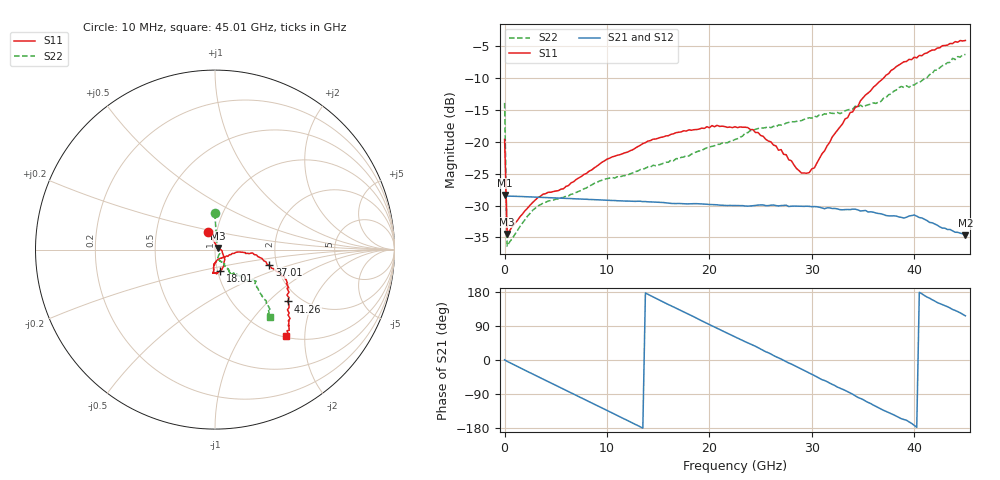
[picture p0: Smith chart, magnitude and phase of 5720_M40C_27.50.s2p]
! Device:  ADRF5720
! Description: 0.5dB LSB GaAs MMIC 6-bit Digital Attenuator
! Frequency:  0.000009 -  40 GHz
! Ports:
!	RF1	= Port 1
!	RF2	= Port 2
! Vdd:  3.3 Volt
! Vss:  -3.3 Volt
! Control:  0/3.3 Volt
! State:  27.50 dB attenuation
! Data:  The device was measured using G-S-G Probes on a matrix board.
!  Data was collected using an calibrated 4 port network analyzer.
!  The reference plane for this measurement is at the launchers.
! Note:  Analog Devices supplies this data as a sample of measured data
!  for this product.  Your particular data for this product may vary.
!  Data was taken at -40 degrees C.
!  Analog Devices reserves the right to change this data at anytime.
# GHZ S DB R 45.0
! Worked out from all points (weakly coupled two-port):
!   181 points, 10 MHz to 45.01 GHz, reference 45 ohm
!   highest |S21| = -28.34 dB at 10 MHz (marker M1); lowest = -34.7 dB at 45.01 GHz (marker M2)
!   lowest |S11| = -34.5 dB at 260 MHz (marker M3), VSWR 1.04, Z = 46.5 + j0.897 ohm
!   |S11| at or under -10 dB: start of sweep to 37.03 GHz
!   |S22| runs from -36.4 to -6.3 dB; largest |S21 - S12| = 0.00019
!   S11 on the Smith chart (normalised r, x): 10 MHz: 0.91, +0.18; 18.01 GHz: 1.03, -0.25; 37.01 GHz: 1.83, -0.35; 41.26 GHz: 1.72, -1.32; 45.01 GHz: 1.02, -1.61
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0.01  -19.62 111.1  -28.34 0.5  -28.36 0.5  -13.90 90.4
0.26  -34.47 30.7  -28.52 -3.6  -28.54 -3.7  -36.38 33.1
2.01  -30.80 3.1  -28.62 -27.2  -28.64 -27.2  -32.16 -18.8
3.26  -28.75 -5.7  -28.70 -43.8  -28.72 -43.8  -30.04 -32.1
5.76  -27.37 -19.7  -28.86 -76.8  -28.88 -76.8  -28.75 -52.0
7.76  -25.12 -33.4  -29.01 -103.2  -29.02 -103.3  -27.38 -65.8
10.01  -22.72 -43.3  -29.18 -133.1  -29.20 -133.1  -25.79 -69.9
15.26  -19.30 -65.5  -29.50 156.3  -29.52 156.3  -23.54 -67.3
18.01  -18.12 -76.6  -29.74 120.4  -29.76 120.3  -22.23 -62.1
22.76  -17.78 -94.6  -30.01 57.9  -30.04 57.8  -19.51 -58.9
24.76  -18.54 -93.3  -29.93 32.6  -29.95 32.5  -17.92 -56.0
27.01  -21.23 -91.8  -30.01 2.7  -30.04 2.5  -17.37 -57.5
29.01  -24.91 -73.5  -30.12 -24.1  -30.14 -24.2  -16.67 -57.4
30.26  -24.10 -41.2  -30.17 -41.0  -30.19 -41.2  -15.97 -56.9
33.26  -16.42 -5.5  -30.64 -80.1  -30.66 -80.2  -15.14 -51.7
37.01  -10.03 -15.9  -31.42 -132.7  -31.43 -132.8  -13.18 -45.1
37.76  -8.80 -19.5  -31.63 -141.5  -31.66 -141.6  -12.51 -44.7
38.76  -7.71 -21.2  -31.86 -155.0  -31.86 -155.1  -11.31 -40.1
40.01  -6.72 -27.2  -31.49 -172.4  -31.50 -172.5  -11.09 -38.5
41.26  -6.06 -35.4  -32.36 166.1  -32.38 166.0  -9.95 -42.0
43.76  -4.59 -45.7  -33.97 133.3  -34.00 133.1  -6.90 -47.4
45.01  -4.10 -50.6  -34.68 116.6  -34.70 116.5  -6.31 -50.6
